(* Logix 5000 DataType export RTA_STRING_4096; software revision 20.01 *)

TYPE RTA_STRING_4096 :   // string type; String Data Type with up to 4096 characters available
STRUCT
   LEN : DINT;
   DATA : SINT[4096];
END_STRUCT
END_TYPE
